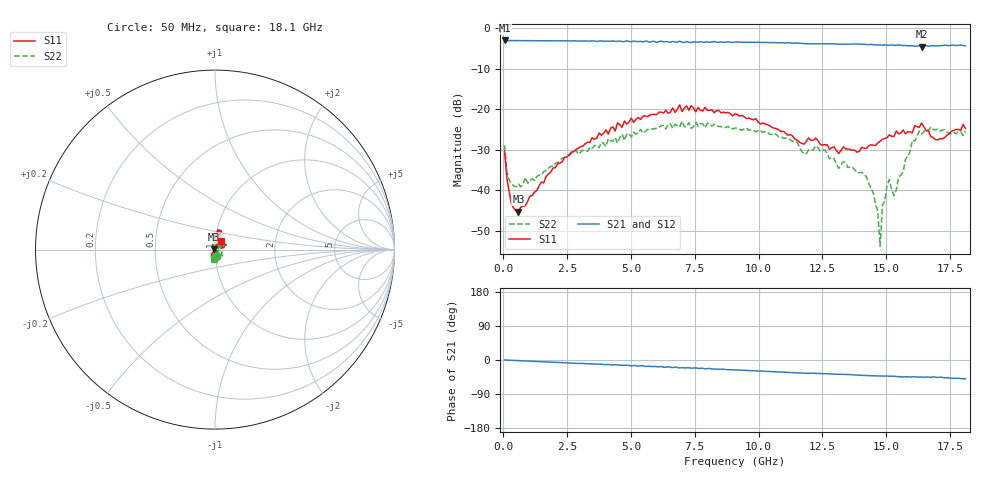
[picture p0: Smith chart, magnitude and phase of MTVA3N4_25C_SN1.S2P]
! Network Analyzer HP8720D.06.14 Serial No. US36140669
! 27 Jun 2005  09:20:06
! Frequency  S11  S21  S12  S22
# HZ  S  DB R 50
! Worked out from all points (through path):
!   201 points, 50 MHz to 18.1 GHz, reference 50 ohm
!   highest |S21| = -3.06 dB at 50 MHz (marker M1); lowest = -4.6 dB at 16.39 GHz (marker M2)
!   group delay of S21, straight-line fit = 7.66 ps
!   lowest |S11| = -45.3 dB at 591.5 MHz (marker M3), VSWR 1.01, Z = 49.5 + j0.12 ohm
!   |S11| at or under -10 dB: start of sweep to end of sweep
!   |S22| runs from -53.8 to -22.9 dB; largest |S21 - S12| = 0.02
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5e7  -30.39 -91.4  -3.06 0.0  -3.08 0.5  -28.95 -81.7
1.4025e8  -37.05 -107.6  -3.13 -0.3  -3.11 -0.2  -35.59 -123.2
3.2075e8  -43.52 -138.7  -3.08 -0.8  -3.10 -0.8  -38.50 -153.7
5.915e8  -45.26 167.2  -3.09 -1.7  -3.12 -1.7  -38.48 179.1
1.94525e9  -34.52 83.8  -3.15 -5.8  -3.15 -5.8  -34.07 118.8
3.1185e9  -29.11 74.0  -3.19 -9.1  -3.21 -9.3  -30.12 108.7
6.09675e9  -20.77 73.1  -3.33 -17.9  -3.27 -17.8  -24.52 71.4
9.075e9  -21.18 86.6  -3.47 -26.1  -3.46 -26.2  -24.67 37.9
1.21435e10  -27.68 87.2  -3.90 -34.7  -3.88 -35.0  -29.95 41.6
1.259475e10  -28.75 75.4  -3.90 -36.1  -3.88 -36.1  -30.05 36.5
1.313625e10  -30.94 65.4  -3.98 -37.6  -3.95 -37.9  -34.60 29.3
1.3407e10  -29.79 57.9  -3.97 -38.1  -3.96 -38.3  -33.15 23.1
1.421925e10  -29.68 20.2  -4.08 -40.6  -4.07 -40.8  -36.66 -68.9
1.46705e10  -28.34 15.4  -4.14 -42.1  -4.15 -42.1  -45.30 -114.1
1.476075e10  -27.91 19.4  -4.20 -42.0  -4.23 -42.6  -53.79 -30.6
1.4851e10  -27.46 19.2  -4.23 -42.4  -4.17 -42.3  -43.54 25.2
1.512175e10  -26.32 16.9  -4.23 -42.9  -4.16 -42.7  -37.38 -31.2
1.530225e10  -26.75 13.7  -4.27 -42.9  -4.19 -43.9  -41.32 -44.2
1.602425e10  -25.85 26.7  -4.36 -44.5  -4.51 -45.6  -27.63 -20.8
1.638525e10  -23.43 21.6  -4.57 -45.0  -4.37 -45.1  -26.12 -44.4
1.692675e10  -27.52 33.6  -4.40 -45.2  -4.28 -45.0  -25.03 -73.4
1.81e10  -24.71 54.9  -4.40 -49.5  -4.36 -50.4  -25.32 -97.5
